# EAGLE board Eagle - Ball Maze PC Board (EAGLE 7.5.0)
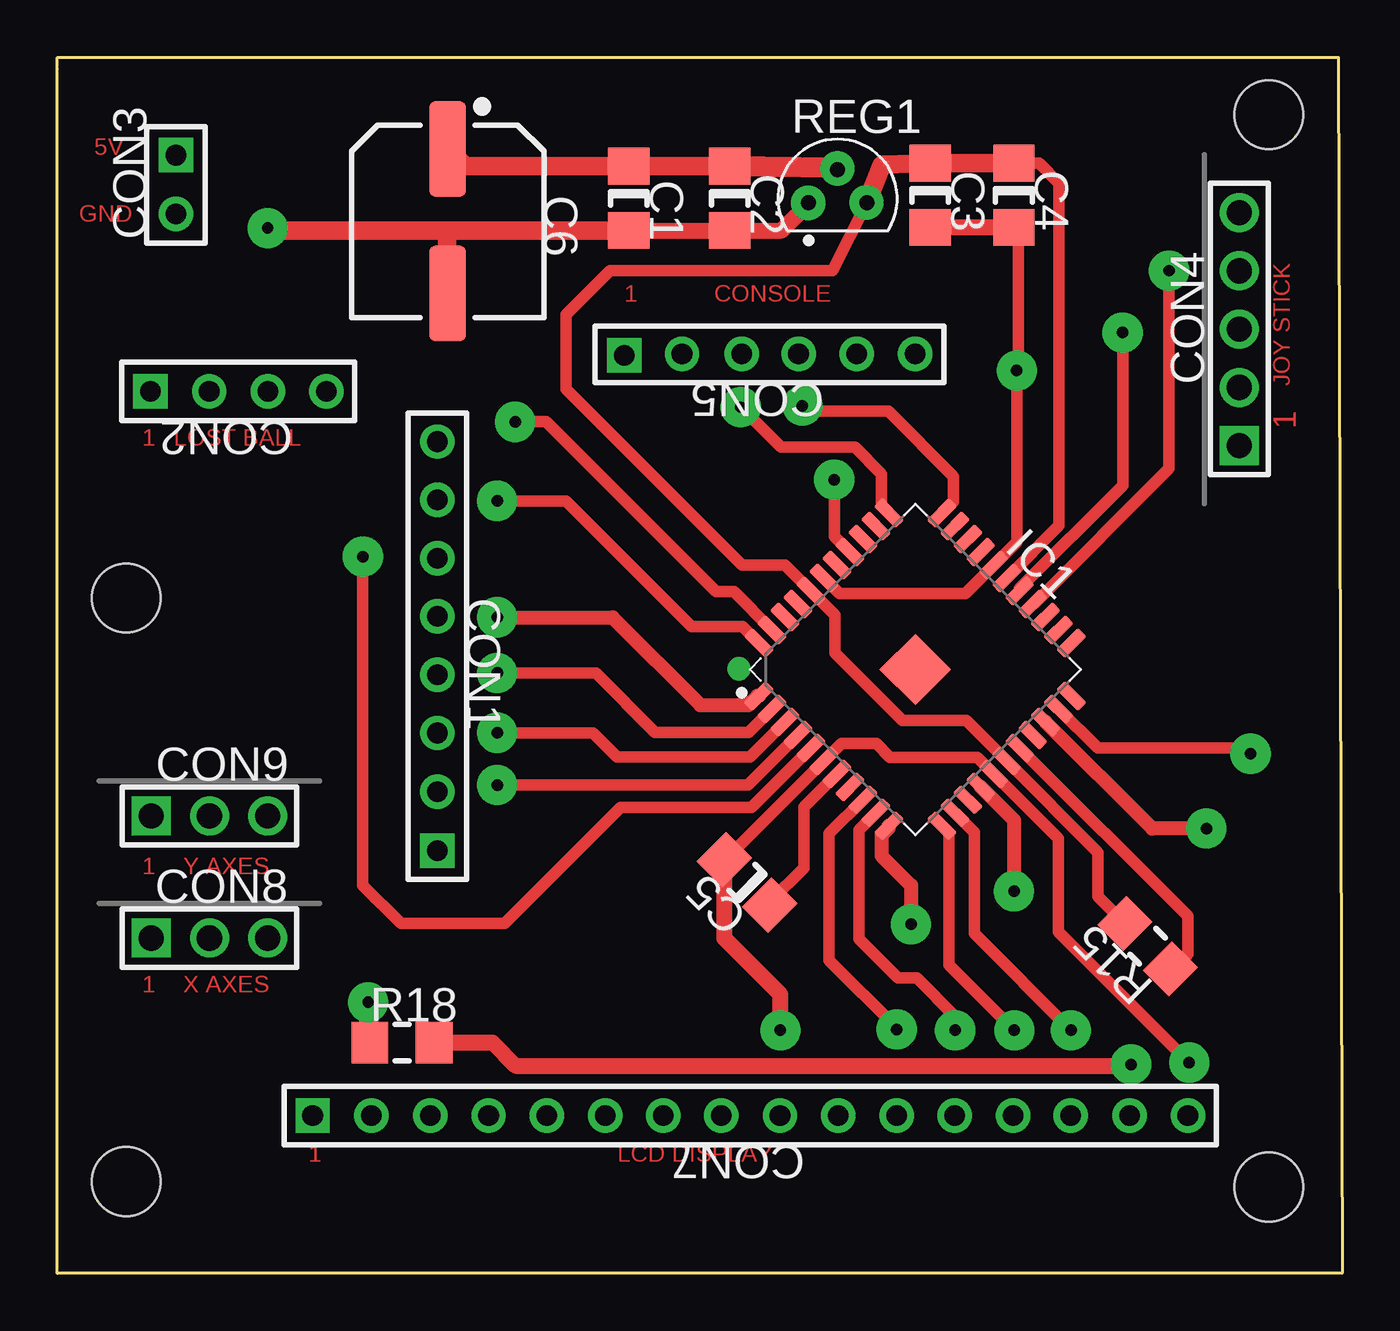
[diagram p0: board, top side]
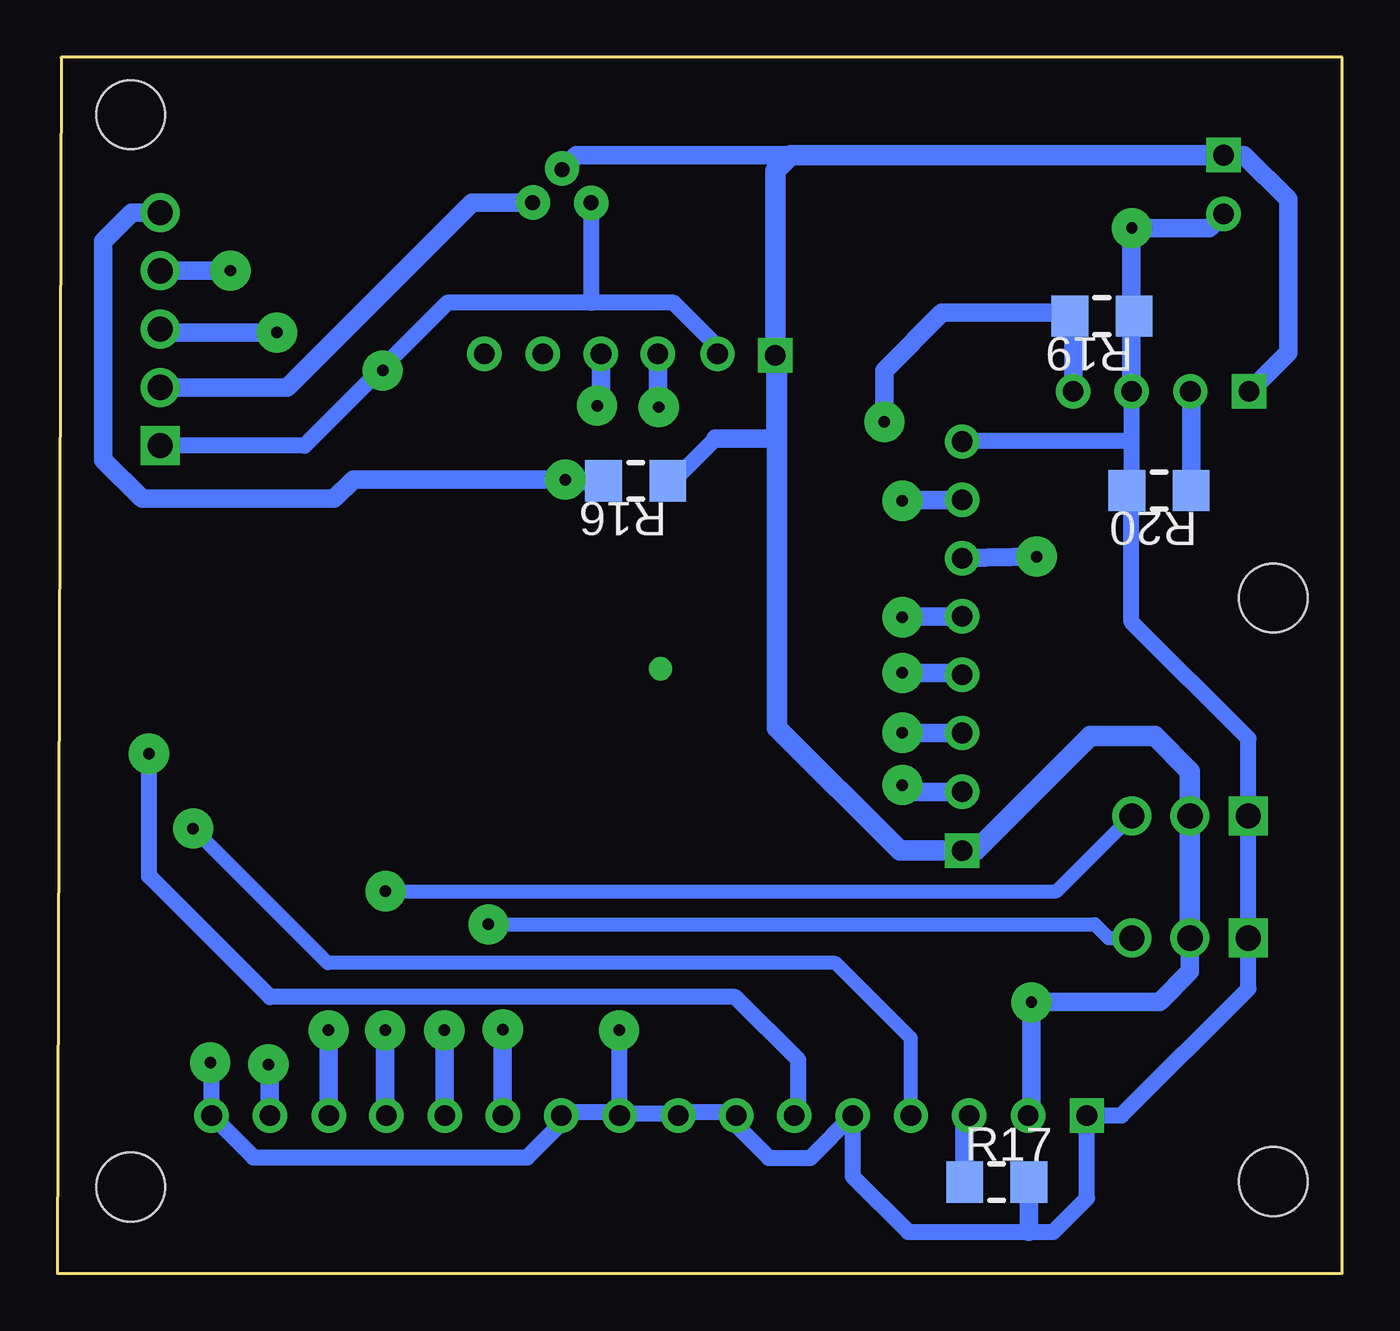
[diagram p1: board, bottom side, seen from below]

Size 56 x 53 mm. Coordinates in mm from the lower left corner, seen from the top.
Outline: 0,53 55.84,53 56,0 0,0 0,52.5 0,53
Copper layers (1*16): Top 0.035mm / dielectric 1.5mm / Bottom 0.035mm
Design rules "default *": minimum track width 10mil, minimum drill 0.61mm, track to track 8mil, track to pad 8mil, pad to pad 8mil, via to via 8mil, smd to smd 8mil, copper to edge 40mil, drill to drill 8mil, minimum pad ring 0mil, minimum via ring 8mil, stop-mask expansion 2mil, vias tented up to drill 20mil, thermal gap 10mil
Net classes: 0 Default: width 0.8 mm, clearance 0.33 mm
Holes 3 mm at 3,4 52.81,3.76 52.8,50.5 3,29.44

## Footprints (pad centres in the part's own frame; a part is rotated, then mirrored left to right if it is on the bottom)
CAP_1206 = smd 1.6 x 1.8: 1 -1.4,0; 2 1.4,0
CAPAE-8.35x8.35h6.2 = smd 4.15 x 1.6: 1 -3.15,0; 2 3.15,0
CON8M = drill 0.9 pad 1.5 square: 1 0,5.105 | drill 0.9 pad 1.5: 2 0,2.54; 3 0,-0.025; 4 0,-2.565; 5 0,-5.105; 6 0,-7.645; 7 0,-10.185; 8 0,-12.725
CON4M = drill 0.9 pad 1.5 square: 1 0,3.835 | drill 0.9 pad 1.5: 2 0,1.27; 3 0,-1.295; 4 0,-3.835
CON2M = drill 0.9 pad 1.5 square: 1 0,2.565 | drill 0.9 pad 1.5: 2 0,0
HDR-1x5T/2.54/12x2 = drill 1.1 pad 1.7 square: 1 -5.08,0 | drill 1.1 pad 1.7: 2 -2.54,0; 3 0,0; 4 2.54,0; 5 5.08,0
CON6F = drill 0.9 pad 1.5 square: 1 -0.033,6.339 | drill 0.9 pad 1.5: 2 0.033,3.821; 3 0.033,1.217; 4 0.033,-1.259; 5 0.033,-3.799; 6 0.033,-6.339
CON16M = drill 0.9 pad 1.5 square: 1 0,19.075 | drill 0.9 pad 1.5: 2 0,16.51; 3 0,13.945; 4 0,11.405; 5 0,8.865; 6 0,6.325; 7 0,3.785; 8 0,1.27; 9 0,-1.295; 10 0,-3.835; 11 0,-6.375; 12 0,-8.915; 13 0,-11.455; 14 0,-13.97; 15 0,-16.535; 16 0,-19.075
HDR-1x3T/2.54/7x2 = drill 1.1 pad 1.7 square: 1 -2.54,0 | drill 1.1 pad 1.7: 2 0,0; 3 2.54,0
QFP45P80_1200X1200X160L60X37T220L = smd 0.55 x 1.36: 1 -4,-5.63; 2 -3.2,-5.63; 3 -2.4,-5.63; 4 -1.6,-5.63; 5 -0.8,-5.63; 6 0,-5.63; 7 0.8,-5.63; 8 1.6,-5.63; 9 2.4,-5.63; 10 3.2,-5.63; 11 4,-5.63; 23 4,5.63; 24 3.2,5.63; 25 2.4,5.63; 26 1.6,5.63; 27 0.8,5.63; 28 0,5.63; 29 -0.8,5.63; 30 -1.6,5.63; 31 -2.4,5.63; 32 -3.2,5.63; 33 -4,5.63 | smd 1.36 x 0.55: 12 5.63,-4; 13 5.63,-3.2; 14 5.63,-2.4; 15 5.63,-1.6; 16 5.63,-0.8; 17 5.63,0; 18 5.63,0.8; 19 5.63,1.6; 20 5.63,2.4; 21 5.63,3.2; 22 5.63,4; 34 -5.63,4; 35 -5.63,3.2; 36 -5.63,2.4; 37 -5.63,1.6; 38 -5.63,0.8; 39 -5.63,0; 40 -5.63,-0.8; 41 -5.63,-1.6; 42 -5.63,-2.4; 43 -5.63,-3.2; 44 -5.63,-4 | smd 2.2 x 2.2: 45 0,0
RES_1206 = smd 1.6 x 1.8: 1 -1.4,0; 2 1.4,0
RES_1206_R16 = smd 1.6 x 1.8: 1 -1.4,0; 2 1.4,0
TO92-127P520H787-3_AP3_STA = drill 0.65 pad 1.05: 1 -1.27,-1.04; 2 0,0.405; 3 1.27,-1.04

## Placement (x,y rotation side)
C1  10uF  [CAP_1206]  24.91,46.85 270 top
C2  100n  [CAP_1206]  29.3,46.85 270 top
C3  10uF  [CAP_1206]  38.04,46.99 270 top
C4  100n  [CAP_1206]  41.69,46.99 270 top
C5  47uF 16V X5R  [CAP_1206]  30.06,17.04 135 top
C6  C220UF  [CAPAE-8.35x8.35h6.2]  17.01,45.86 270 top
CON1  51022-0800  [CON8M]  16.57,23.53 180 top
CON2  51022-0400  [CON4M]  7.89,38.44 90 top
CON3  DF4-2P-2C  [CON2M]  5.17,46.17 0 top
CON4  644456-5  [HDR-1x5T/2.54/12x2]  51.52,41.16 90 top
CON5  C:\Program Files\DipTrace\models3d\Con Headers\Part 2\hdrf-1x6t_2.54_16x3.step  [CON6F]  31.05,40.04 90 top
CON7  HDRF-1X16  [CON16M]  30.2,6.88 90 top
CON8  644456-3  [HDR-1x3T/2.54/7x2]  6.63,14.61 0 top
CON9  644456-3  [HDR-1x3T/2.54/7x2]  6.63,19.93 0 top
IC1  PIC32MX-D/A 44PINS  [QFP45P80_1200X1200X160L60X37T220L]  37.4,26.32 315 top
R15  10K  [RES_1206]  47.52,14.26 135 top
R16  1K  [RES_1206_R16]  30.79,34.54 180 bottom
R17  1K8  [RES_1206_R16]  15.06,3.98 360 bottom
R18  1K8  [RES_1206]  15.02,10.06 0 top
R19  10K  [RES_1206_R16]  10.47,41.72 180 bottom
R20  150R  [RES_1206_R16]  7.98,34.12 180 bottom
REG1  MCP1700T-33  [TO92-127P520H787-3_AP3_STA]  34.01,47.7 0 top

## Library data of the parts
C1 C3 C5 C6 CON7 IC1 R15-R20 = common
C2 C4 = common; DESCRIPTION: Non-polarized
CON1 CON2 CON5 = common; DATASHEET: http://datasheets.diptrace.com/con_board_in/510221400_sd.pdf; MANUFACTURER: Molex
CON3 = common; DATASHEET: http://datasheets.diptrace.com/con_board_in/DF4.pdf; MANUFACTURER: Hirose
CON4 CON8 CON9 = common; DATASHEET: http://datasheets.diptrace.com/con_headers/ENG_CD_644456_D2.pdf; MANUFACTURER: TE Connectivity
REG1 = common; DATASHEET: http://datasheets.diptrace.com/microchip/20001826d.pdf; MANUFACTURER: Microchip; PART_NUMBER_(DIGI-KEY): MCP1700T3302EMBDKR-ND; UNIQUE_NAME: MICROCHIP_C04-029C

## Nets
D4: CON7.11 IC1.9
D5: CON7.12 IC1.10
D6: CON7.13 IC1.12
D7: CON7.14 IC1.13
EN: CON7.6 IC1.21
Net_0: C1.2 C2.2 C3.2 C4.2 C5.2 C6.2 CON1.8 CON2.3 CON3.2 CON4.1 CON5.2 CON7.1 CON7.5 CON7.7 CON7.8 CON7.9 CON7.10 CON7.16 CON8.1 CON9.1 IC1.6 IC1.16 IC1.29 IC1.39 R17.2 R19.1 R20.2 REG1.1
Net_1: C3.1 C4.1 CON4.2 IC1.17 IC1.28 IC1.40 R15.2 REG1.3
Net_2: CON4.4 IC1.26
Net_4: C1.1 C2.1 C6.1 CON1.1 CON2.1 CON3.1 CON5.1 CON7.2 CON8.2 CON9.2 R16.1 R18.1 REG1.2
Net_14: CON5.3 IC1.34
Net_16: CON5.4 IC1.33
Net_22: CON7.3 R17.1
Net_23: CON4.3 IC1.27
Net_24: IC1.18 R15.1
Net_27: C5.1 IC1.7
Net_29: CON4.5 IC1.37 R16.2
Net_31: CON2.2 R20.1
Net_36: CON7.15 R18.2
Net_42: CON9.3 IC1.15
Net_43: CON8.3 IC1.11
Opto1: CON1.2 IC1.4
Opto2: CON1.3 IC1.3
Opto3: CON1.4 IC1.2
Opto4: CON1.5 IC1.1
Opto5: CON1.6 IC1.5
OptoFIN: CON1.7 IC1.44
OptoLOST: CON2.4 IC1.43 R19.2
RS: CON7.4 IC1.20

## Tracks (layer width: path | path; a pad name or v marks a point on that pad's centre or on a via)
D4  (via drill 0.5 pad 1.75)
  Top 0.5: IC1.9 33.63,19.16 33.63,13.64 36.59,10.69 v36.59,10.63
  Bottom 0.8: v36.59,10.63 CON7.11
D5  (via drill 0.5 pad 1.75)
  Top 0.5: v39.13,10.59 39.13,11.21 37.47,12.87 36.65,12.87 34.94,14.58 34.94,19.34 IC1.10
  Bottom 0.8: v39.13,10.59 39.13,7.23 39.12,7.21 CON7.12
D6  (via drill 0.5 pad 1.75)
  Top 0.5: v41.71,10.59 38.86,13.45 38.86,19.2 IC1.12
  Bottom 0.8: v41.71,10.59 41.71,7.45 41.66,7.39 CON7.13
D7  (via drill 0.5 pad 1.75)
  Top 0.5: v44.18,10.59 39.97,14.8 39.97,19.22 IC1.13
  Bottom 0.8: v44.18,10.59 44.18,7.52 44.17,7.51 CON7.14
EN  (via drill 0.5 pad 1.75)
  Top 0.5: v52.01,22.65 52.01,22.89 45.35,22.89 IC1.21
  Bottom 0.7: CON7.6 23.71,7.05 23.71,9.29 26.46,12.05 46.73,12.05 52.01,17.32 v52.01,22.65
Net_0  (via drill 0.5 pad 1.5, 0.5 pad 1.75)
  Top 0.5: C5.2 29.1,18.03 IC1.6 34.17,23.09 35.69,23.09 36.3,22.49 40.09,22.49 IC1.16 43.63,18.95 43.63,14.88 v49.34,9.18 | IC1.39 34.09,29.63 39.57,29.63 IC1.29 41.82,31.88 41.82,39.08 41.89,39.02 41.89,39.35 41.89,45.39 C4.2
  Top 0.7: v31.52,10.59 31.52,12.15 29.07,14.6 C5.2 | C4.2 C3.2 | C3.2 | C2.2 31.57,45.45 32.74,46.62 REG1.1 | C1.2 C2.2 | C2.2
  Top 0.8: C1.2 16.98,45.45 | 16.98,45.45 9.17,45.45 v9.17,45.56 | C6.2 16.98,42.71 16.98,45.45 | v41.82,39.35 41.89,39.35
  Bottom 0.7: CON7.9 31.5,6.97 28.93,6.97 CON7.8 28.93,7.04 26.42,7.04 CON7.7 26.42,6.46 24.99,5.03 23.18,5.03 CON7.5 21.34,4.23 18.91,1.8 13.66,1.8 12.59,1.8 11.13,3.27 CON7.1 9.62,6.88 4.09,12.4 CON8.1 CON9.1 4.09,23.3 9.18,28.39 9.18,33.91 R20.2 9.18,34.32 9.18,36.27 | CON7.9 31.5,7.04 34.04,7.04 CON7.10 34.04,6.54 35.52,5.05 47.45,5.05 CON7.16 49.28,9.12 v49.34,9.18 | v31.52,10.59 31.52,6.89 CON7.9 | CON2.3 9.18,36.27 | 9.18,36.27 16.57,36.27 CON1.8 | CON5.2 27.23,40.39 29.14,42.31 32.72,42.31 | 32.72,42.31 32.72,46.63 | 32.72,46.63 32.74,46.63 REG1.1 | 32.72,42.31 39,42.31 41.89,39.41 | 41.89,39.41 45.23,36.08 CON4.1 | v41.82,39.35 41.89,39.41 | v32.73,46.66 32.72,46.63
  Bottom 0.8: CON2.3 9.18,41.83 | 9.18,41.83 9.18,45.54 v9.17,45.56 5.79,45.56 CON3.2 | 9.18,41.83 R19.1 | R17.2 13.66,1.8
Net_1  (via drill 0.5 pad 1.5)
  Top 0.5: REG1.3 33.79,43.7 24.08,43.7 22.17,41.79 22.17,38.53 29.84,30.86 31.72,30.86 IC1.40 33.9,28.68 33.9,27.04 36.84,24.1 39.62,24.1 IC1.17 45.36,18.35 45.36,16.42 R15.2 | IC1.28 43.66,32.59 43.66,47.52 42.8,48.39 C4.1
  Top 0.8: REG1.3 | REG1.3 35.95,48.32 C3.1 | C4.1 C3.1 | C3.1 | v35.27,46.68 REG1.3
  Bottom 0.8: REG1.3 37.93,46.66 45.98,38.62 CON4.2
Net_2  (via drill 0.5 pad 1.75)
  Top 0.5: IC1.26 42.56,29.17 48.45,35.07 v48.45,43.7
  Bottom 0.8: v48.45,43.7 CON4.4
Net_4  (via drill 0.5 pad 1.5, 0.5 pad 1.75)
  Top 0.8: v13.55,11.81 13.55,10.06 R18.1 | C2.1 C1.1 | C1.1 | C1.1 17.77,48.25 C6.1
  Top 0.9: REG1.2 | REG1.2 33.99,48.19 | 33.99,48.19 C2.1 | v34,48.15 33.99,48.19
  Bottom 0.7: R16.1 29.17,34.54 27.32,36.39
  Bottom 0.8: CON8.2 6.63,13.15 7.95,11.83 13.53,11.83 v13.55,11.81 13.55,7.02 CON7.2 | CON2.1 2.35,40.14 2.35,46.81 4.28,48.74 CON3.1 33.38,48.74 REG1.2 | 27.32,36.39 24.71,36.39 CON5.1
  Bottom 0.9: CON3.1 24.02,48.74 24.71,48.06 CON5.1 24.62,39.92 24.62,23.77 19.27,18.42 CON1.1 15.96,18.42 10.97,23.41 8.17,23.41 6.63,21.87 CON9.2 CON8.2
Net_14  (via drill 0.5 pad 1.75)
  Top 0.5: v29.79,37.76 31.54,36 34.76,36 35.92,34.83 35.92,33.45 IC1.34
  Bottom 0.8: CON5.3 29.83,37.8 v29.79,37.76
Net_16  (via drill 0.5 pad 1.75)
  Top 0.5: v32.48,37.81 32.71,37.58 36.22,37.58 39.06,34.74 39.06,33.64 IC1.33
  Bottom 0.8: CON5.4 32.31,37.98 v32.48,37.81
Net_22
  Bottom 0.8: R17.1 16.46,6.88 CON7.3
Net_23  (via drill 0.5 pad 1.75)
  Top 0.5: IC1.27 41.94,29.85 46.43,34.34 v46.43,41
  Bottom 0.8: v46.43,41 51.37,41 CON4.3
Net_24
  Top 0.5: R15.1 48.64,13.27 49.27,13.9 49.27,15.58 IC1.18
Net_27
  Top 0.5: IC1.7 32.54,20.33 32.54,17.68 31.05,16.19 C5.1
Net_29  (via drill 0.5 pad 1.75)
  Top 0.5: IC1.37 33.86,32.11 v33.86,34.59
  Bottom 0.8: v33.86,34.59 | v33.86,34.59 33.88,34.54 R16.2 | CON4.5 52.76,46.24 54,44.99 54,35.46 52.31,33.76 43.93,33.76 43.09,34.59 v33.86,34.59
Net_31
  Bottom 0.8: R20.1 6.58,38.41 CON2.2
Net_36  (via drill 0.5 pad 1.75)
  Top 0.7: R18.2 18.96,10.06 19.98,9.04 46.8,9.04 v46.8,9.1
  Bottom 0.8: CON7.15 46.74,9.04 v46.8,9.1
Net_42  (via drill 0.5 pad 1.75)
  Top 0.6: IC1.15 41.7,19.75 v41.7,16.65
  Bottom 0.6: v41.7,16.65 12.45,16.65 CON9.3
Net_43  (via drill 0.5 pad 1.75)
  Top 0.6: IC1.11 36.24,19.41 35.92,19.09 35.92,18.2 37.21,16.91 v37.21,15.21
  Bottom 0.6: v37.21,15.21 10.78,15.21 10.18,14.61 CON8.3
Opto1  (via drill 0.5 pad 1.75)
  Top 0.5: v19.17,21.29 30.1,21.29 IC1.4
  Bottom 0.8: v19.17,21.29 18.99,21.29 18.69,20.99 CON1.2
Opto2  (via drill 0.5 pad 1.75)
  Top 0.5: v19.17,23.56 23.35,23.56 24.4,22.51 30.19,22.51 IC1.3
  Bottom 0.8: v19.17,23.56 17.74,23.56 17.73,23.55 CON1.3
Opto3  (via drill 0.5 pad 1.75)
  Top 0.5: IC1.2 30.13,23.58 26.05,23.58 23.47,26.17 v19.17,26.17
  Bottom 0.8: v19.17,26.17 16.97,26.17 16.9,26.09 CON1.4
Opto4  (via drill 0.5 pad 1.75)
  Top 0.6: v19.17,28.59 24.2,28.59 28.03,24.76 30.11,24.76 30.51,25.17 IC1.1
  Bottom 0.8: CON1.5 19.13,28.63 v19.17,28.59
Opto5  (via drill 0.5 pad 1.75)
  Top 0.5: v13.32,31.23 13.32,16.91 14.98,15.24 19.49,15.24 24.55,20.3 30.25,20.3 IC1.5
  Bottom 0.8: v13.32,31.23 CON1.6
OptoFIN  (via drill 0.5 pad 1.75)
  Top 0.5: v19.17,33.67 22.17,33.67 27.63,28.2 29.86,28.2 IC1.44
  Bottom 0.8: CON1.7 19.12,33.71 v19.17,33.67
OptoLOST  (via drill 0.5 pad 1.75)
  Top 0.5: v19.96,37.12 21.3,37.12 28.71,29.71 29.48,29.71 IC1.43
  Bottom 0.5: R19.2 14.14,41.72 14.29,41.87
  Bottom 0.8: CON2.4 11.72,41.87 14.29,41.87 17.44,41.87 19.96,39.35 v19.96,37.12
RS  (via drill 0.5 pad 1.75)
  Top 0.6: v50.08,19.39 47.72,19.39 IC1.20
  Bottom 0.6: CON7.4 18.8,10.24 22.07,13.52 44.21,13.52 v50.08,19.39
S$1  (via drill 0 pad 1.02)
  other vias: 29.71,26.34

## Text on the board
Top: 5V | GND | 1 | CONSOLE | JOY STICK | 1 | LOST BALL | 1 | 1 | Y AXES | 1 | X AXES | 1 | LCD DISPLAY
tPlace: REG1 | C3 | C4 | C1 | C2 | C6 | CON3 | CON5 | CON4 | CON2 | IC1 | CON1 | CON9 | CON8 | C5 | R15 | R18 | CON7
bPlace: R19 | R20 | R16 | R17
tCream: 5V | GND | LOST BALL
